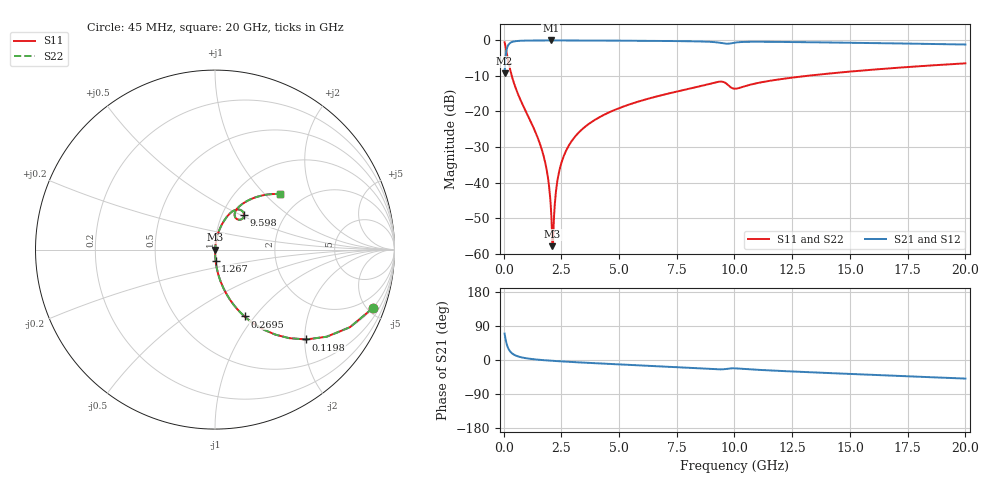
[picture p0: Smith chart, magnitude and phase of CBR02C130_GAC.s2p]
! S-parameter model data by Modelithics Inc.  support@modelithics.com 813-866-6335  Tampa FL USA
! S-Parameter data specifications:
! Substrate: 20-mil Rogers 4350B, substrate thickness, H=0.508mm, Dielectric constant, Er=3.75
! PCB Mounting Pad Footprint: Pad width, PadW=0.32mm , Pad length, PadL=0.37mm , Pad gap, PadG (edge-to-edge)=0.19mm , Reference planes=0.93mm apart
#  GHz  S  MA  R 50
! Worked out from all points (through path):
!   801 points, 45 MHz to 20 GHz, reference 50 ohm
!   highest |S21| = -0.01 dB at 2.041 GHz (marker M1); lowest = -9.2 dB at 45 MHz (marker M2)
!   group delay of S21, straight-line fit = 7.89 ps
!   lowest |S11| = -57.9 dB at 2.115 GHz (marker M3), VSWR 1.00, Z = 50.1 - j0.0683 ohm
!   |S11| at or under -10 dB: 356.2 MHz to 13.11 GHz (12.75 GHz wide, 189 % of centre)
!   |S22| runs from -57.9 to -0.6 dB; largest |S21 - S12| = 0
!   S11 on the Smith chart (normalised r, x): 45 MHz: 1.00, -5.41; 119.8 MHz: 1.00, -2.03; 269.5 MHz: 1.00, -0.89; 1.267 GHz: 1.00, -0.12; 9.598 GHz: 1.26, +0.53; 20 GHz: 1.54, +1.23
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0.045  0.9382 -20.3  0.3458 69.7  0.3458 69.7  0.9382 -20.3
0.119831  0.7126 -44.6  0.7011 45.3  0.7011 45.3  0.7126 -44.6
0.269494  0.4072 -66.2  0.9128 23.8  0.9128 23.8  0.4072 -66.2
0.543875  0.2054 -78.5  0.978 11.3  0.978 11.3  0.2054 -78.5
1.267244  0.06208 -86.9  0.9971 2.3  0.9971 2.3  0.06208 -86.9
1.816006  0.01828 -87.6  0.9988 -0.8  0.9988 -0.8  0.01828 -87.6
1.940725  0.01061 -85.6  0.9988 -1.4  0.9988 -1.4  0.01061 -85.6
2.0405  0.004905 -79.1  0.9989 -1.8  0.9989 -1.8  0.004905 -79.1
2.115331  0.001272 -32.4  0.9989 -2.1  0.9989 -2.1  0.001272 -32.4
2.190163  0.003538 69.2  0.9988 -2.4  0.9988 -2.4  0.003538 69.2
2.289938  0.008567 79.6  0.9988 -2.8  0.9988 -2.8  0.008567 79.6
2.364769  0.01226 81.5  0.9987 -3.1  0.9987 -3.1  0.01226 81.5
2.539375  0.02053 82.9  0.9986 -3.8  0.9986 -3.8  0.02053 82.9
2.888587  0.03581 83.0  0.9981 -5.0  0.9981 -5.0  0.03581 83.0
3.387462  0.05559 82.0  0.9971 -6.7  0.9971 -6.7  0.05559 82.0
4.659594  0.1001 78.6  0.9933 -10.5  0.9933 -10.5  0.1001 78.6
6.704981  0.1651 72.9  0.984 -16.4  0.984 -16.4  0.1651 72.9
9.598456  0.2534 50.3  0.9011 -24.0  0.9011 -24.0  0.2534 50.3
10.0225  0.2092 54.7  0.9309 -22.0  0.9309 -22.0  0.2092 54.7
13.36496  0.323 56.7  0.942 -32.6  0.942 -32.6  0.323 56.7
16.68248  0.4038 48.5  0.9111 -41.0  0.9111 -41.0  0.4038 48.5
20  0.4758 40.6  0.8757 -49.0  0.8757 -49.0  0.4758 40.6
